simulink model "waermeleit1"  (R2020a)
settings: Solver=ode45  StartTime=0.0  StopTime=2000  MaxStep=0.2  RelTol=1e-3  EnableMultiTasking=on
InitFcn:
  | init_waermeleit1
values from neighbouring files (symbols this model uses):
  c1 = 1e7    (= 10000000)    [init_sink.m]    (also in init_waermeleit1.m = 0.002908; init_waermeleit2.m = 0.0727)
  T0 = 500    [init_waermeleit1.m]    (also in init_waermeleit2.m)
  Tl = 300    [init_waermeleit1.m]    (also in init_waermeleit2.m)
  Tr = 250    [init_waermeleit1.m]    (also in init_waermeleit2.m)

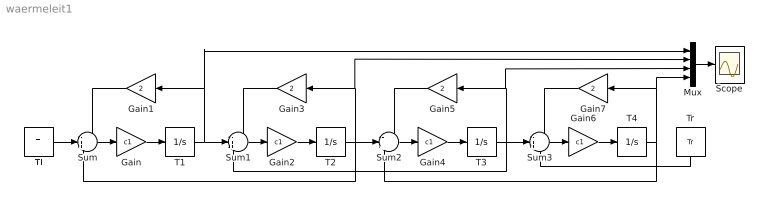
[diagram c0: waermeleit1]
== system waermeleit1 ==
  Gain{,2,4,6} (4 alike) : Gain  Gain=c1
  Gain{1,3,5,7} (4 alike) : Gain  Gain=2
  Mux : Mux
  Scope : Scope
  Sum{,1..3} (4 alike) : Sum  Inputs=-++
  T{1..4} (4 alike) : Integrator  InitialCondition=T0
  Tl : Constant  Value=Tl
  Tr : Constant  Value=Tr
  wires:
  Gain/1 -> T1/1
  Sum/1 -> Gain/1
  T1/1 -> Sum1/2, Gain1/1, Mux/1
  Gain1/1 -> Sum/1
  Gain2/1 -> T2/1
  Sum1/1 -> Gain2/1
  T2/1 -> Sum2/2, Sum/3, Gain3/1, Mux/2
  Gain3/1 -> Sum1/1
  Gain4/1 -> T3/1
  Sum2/1 -> Gain4/1
  T3/1 -> Sum3/2, Sum1/3, Gain5/1, Mux/3
  Gain5/1 -> Sum2/1
  Gain6/1 -> T4/1
  Sum3/1 -> Gain6/1
  T4/1 -> Sum2/3, Gain7/1, Mux/4
  Gain7/1 -> Sum3/1
  Tl/1 -> Sum/2
  Tr/1 -> Sum3/3
  Mux/1 -> Scope/1
